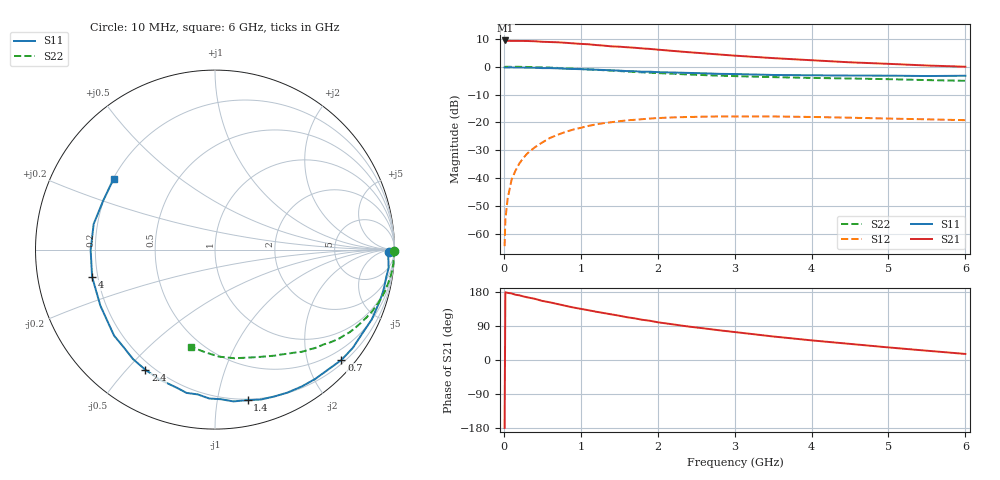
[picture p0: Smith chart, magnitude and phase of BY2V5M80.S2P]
! SIEMENS Small Signal Semiconductors
! BFY420
! Si NPN RF SIEGET Grounded Emitter Transistor in MICRO-X
! VCE = 2.5 V  IC = 0.8 mA
! Common Emitter S-Parameters:  October  1996
# GHz  S  MA  R  50
!  f  S11  S21  S12  S22
! GHz  MAG  ANG  MAG  ANG  MAG  ANG  MAG  ANG
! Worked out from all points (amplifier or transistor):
!   36 points, 10 MHz to 6 GHz, reference 50 ohm
!   highest |S21| = 9.4 dB at 20 MHz (marker M1)
!   |S21| within 3 dB of that: start of sweep to 1.878 GHz
!   unconditionally stable (mu >= 1): 4.637 GHz to end of sweep
!   at 250 MHz: K = 0.04, MSG = 21.1 dB, |S12| = -32.9 dB
!   at 1.4 GHz: K = 0.19, MSG = 13.6 dB, |S12| = -19.9 dB
!   at 6 GHz: K = 1.37, MAG = 5.9 dB, |S12| = -19.2 dB
!   S11 on the Smith chart (normalised r, x): 10 MHz: 58, -24; 700 MHz: 0.27, -2.64; 1.4 GHz: 0.19, -1.22; 2.4 GHz: 0.17, -0.56; 4 GHz: 0.18, -0.11; 6 GHz: 0.20, +0.30
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0.01  0.9709 -0.7  2.952 -179.3  0.0006 88.5  0.9999 -0.3
0.02  0.9663 -1.3  2.96 178.8  0.0018 84.1  0.9952 -0.5
0.05  0.9671 -3.0  2.912 177.2  0.0043 91.1  0.9981 -1.4
0.1  0.973 -6.1  2.908 175.7  0.0093 86.7  0.9938 -2.9
0.15  0.9664 -9.0  2.906 172.3  0.0135 83.0  0.9968 -4.3
0.2  0.9658 -12.2  2.902 170.7  0.0182 82.8  0.995 -5.7
0.4  0.9562 -24.0  2.864 161.6  0.0355 75.6  0.9821 -11.3
0.5  0.944 -29.9  2.803 155.9  0.0437 72.2  0.9739 -14.1
0.7  0.9351 -41.1  2.743 147.6  0.0599 65.3  0.9504 -19.5
0.9  0.9117 -52.2  2.625 138.7  0.0742 57.8  0.9233 -24.4
1.1  0.893 -63.2  2.528 131.3  0.0866 51.7  0.8947 -29.2
1.4  0.8583 -77.8  2.317 120.3  0.101 43.1  0.8517 -35.5
1.7  0.8303 -92.2  2.191 109.9  0.1114 35.4  0.8036 -41.1
2  0.7986 -105.4  2.026 99.6  0.1197 28.3  0.7686 -46.2
2.2  0.7872 -113.0  1.92 94.0  0.123 24.2  0.7483 -49.5
2.4  0.7738 -120.1  1.822 88.3  0.1251 20.9  0.7245 -52.4
2.8  0.7442 -133.4  1.656 78.4  0.128 14.4  0.6902 -57.9
3.5  0.711 -153.9  1.427 62.1  0.1279 5.9  0.6503 -66.7
4  0.7014 -167.5  1.307 51.8  0.1253 1.3  0.6288 -73.2
4.5  0.6928 -179.8  1.199 42.5  0.1215 -2.3  0.6146 -79.9
5.5  0.68 156.3  1.051 24.5  0.1136 -5.3  0.575 -95.3
6  0.6884 145.2  0.999 16.0  0.1097 -4.6  0.5579 -104.0
